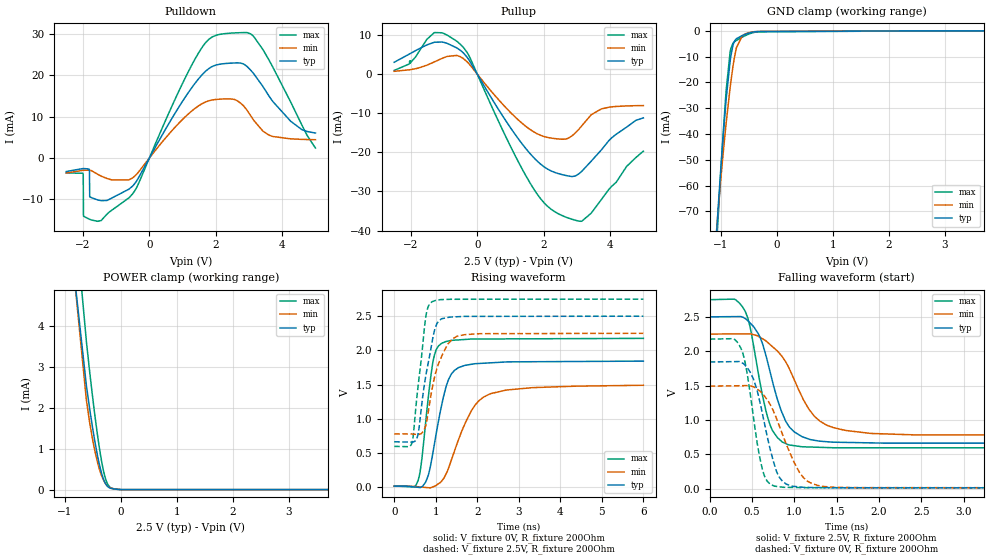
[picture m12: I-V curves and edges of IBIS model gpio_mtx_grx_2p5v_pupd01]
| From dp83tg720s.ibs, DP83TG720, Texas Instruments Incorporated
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[Model]   gpio_mtx_grx_2p5v_pupd01
Model_type   I/O
Polarity   Non-Inverting
Enable   Active-Low
Vinl = 0.75
Vinh = 1.75
Vmeas = 1.25
Vref = 0
Cref = 2pF
Rref = 100000
|   typ   min   max
C_comp   1.19pF   1.18pF   1.2pF
[Voltage Range]   2.5   2.25   2.75
[Temperature Range]   27   150   -40
[Pullup Reference]   2.5   2.25   2.75
[Pulldown Reference]   0   0   0
[Power Clamp Reference]   2.5   2.25   2.75
[GND Clamp Reference]   0   0   0
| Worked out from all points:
|   slope of the pulldown table from 0 to 0.375 V, typ, clamps not added: 69.3 ohm
|   slope of the pullup table from 0 to 0.375 V, typ, clamps not added: 69.5 ohm
|   GND clamp passes 1 mA (typ) near -0.52 V on its own axis
|   POWER clamp passes 1 mA (typ) near -0.44 V on its own axis
|   falling waveform, V_fixture 2.5V, R_fixture 200Ohm: 20-80 % time 264ps typ, 391ps min, 205ps max; typ from 2.5 V to 0.662 V
|   rising waveform, V_fixture 0V, R_fixture 200Ohm: 20-80 % time 357ps typ, 617ps min, 238ps max; typ from 0.013 V to 1.84 V
|   rising waveform, V_fixture 2.5V, R_fixture 200Ohm: 20-80 % time 286ps typ, 362ps min, 225ps max; typ from 0.662 V to 2.5 V
|   falling waveform, V_fixture 0V, R_fixture 200Ohm: 20-80 % time 208ps typ, 303ps min, 161ps max; typ from 1.84 V to 0.013 V
[Pulldown]
|   Voltage   I(typ)   I(min)   I(max)
-2.5V     -3.265mA   -3.621mA   -3.605mA
-2.005V   -2.554mA   -2.975mA   -3.687mA
-1.99V    -2.541mA   -2.964mA   -3.987mA
-1.982V   -2.535mA   -2.958mA   -14.07mA
-1.802V   -2.906mA   -2.952mA   -14.82mA
-1.795V   -9.394mA   -2.961mA   -14.85mA
-1.788V   -9.424mA   -2.97mA    -14.87mA
-617.5mV  -7.551mA   -5.289mA   -9.664mA
1.482V    19.21mA    12.66mA    25.49mA
2.322V    22.93mA    14.34mA    30.18mA
3.147V    20.37mA    9.1mA      29.38mA
5V        6.062mA    4.441mA    2.42mA
[GND Clamp]
|   Voltage   I(typ)   I(min)   I(max)
-2.5V     -617.9mA   -534.4mA   -681.3mA
-1.097V   -85.38mA   -83.09mA   -91.27mA
-1.038V   -65.28mA   -66.86mA   -68.32mA
-962.5mV  -41.99mA   -48.38mA   -41.28mA
-917.5mV  -29.66mA   -38.4mA    -26.83mA
-835mV    -11.96mA   -22.23mA   -8.453mA
-782.5mV  -5.504mA   -13.69mA   -4.805mA
-722.5mV  -3.044mA   -6.63mA    -3.739mA
-617.5mV  -1.829mA   -1.936mA   -2.464mA
-565mV    -1.375mA   -1.221mA   -1.889mA
-302.5mV  -289.6uA   -223.3uA   -396.9uA
5V        0A         0A         0A
[Pullup]
|   Voltage   I(typ)   I(min)   I(max)
-2.5V     3.036mA    720.5uA    942.2uA
-2.042V   5.137mA    1.103mA    2.614mA
-1.3V     8.128mA    3.091mA    10.57mA
-617.5mV  6.711mA    4.78mA     8.425mA
-250mV    3.626mA    2.646mA    4.708mA
852.5mV   -11.84mA   -8.504mA   -15.89mA
1.7V      -21.35mA   -14.76mA   -29.37mA
2.217V    -24.74mA   -16.36mA   -34.52mA
2.848V    -26.19mA   -15.81mA   -37.11mA
3.147V    -24.84mA   -13.2mA    -37.61mA
3.732V    -19.41mA   -8.91mA    -32.11mA
5V        -11.19mA   -8.043mA   -19.7mA
[POWER Clamp]
|   Voltage   I(typ)   I(min)   I(max)
-2.5V     97.53mA    60.54mA    150.4mA
-1.09V    8.453mA    8.804mA    10.81mA
-617.5mV  2.546mA    2.188mA    3.625mA
-565mV    2.037mA    1.696mA    2.964mA
-505mV    1.499mA    1.216mA    2.252mA
-422.5mV  855.7uA    690.1uA    1.37mA
-370mV    524.7uA    436.5uA    888.5uA
-325mV    305.8uA    271.3uA    544.9uA
-280mV    156.5uA    154.6uA    285.8uA
-197.5mV  39.48uA    47.14uA    60.64uA
12.5mV    0A         0A         0A
5V        0A         0A         0A
[Ramp]
R_load = 200
|   typ   min   max
dV/dt_r   1.09795/3.56346e-10   0.886285/6.13825e-10   1.2967/2.36701e-10
dV/dt_f   1.10266/2.61664e-10   0.884047/3.89939e-10   1.29322/2.04854e-10
[Falling Waveform]
V_fixture = 2.5V
V_fixture_min = 2.25V
V_fixture_max = 2.75V
R_fixture = 200Ohm
C_fixture = 0F
|   Time   V(typ)   V(min)   V(max)
0s        2.5V       2.25V      2.75V
289.7ps   2.503V     2.252V     2.758V
411.7ps   2.481V     2.252V     2.599V
476.7ps   2.411V     2.253V     2.355V
581.8ps   2.237V     2.212V     1.629V
702.2ps   1.754V     2.109V     967.7mV
929ps     921mV      1.774V     639.2mV
1.239ns   703.9mV    1.052V     604mV
1.618ns   673mV      845.1mV    595.4mV
6ns       662.2mV    776.4mV    594.6mV
[Rising Waveform]
V_fixture = 0V
V_fixture_min = 0V
V_fixture_max = 0V
R_fixture = 200Ohm
C_fixture = 0F
|   Time   V(typ)   V(min)   V(max)
0s        12.69mV    11.93mV    14.4mV
573ps     -4.336mV   3.092mV    91.58mV
661.7ps   2.918mV    -1.788mV   389.7mV
762.6ps   78.23mV    -7.336mV   976.7mV
926.7ps   482.4mV    840.7uV    1.81V
1.14ns    1.188V     83.97mV    2.102V
1.451ns   1.707V     524.7mV    2.149V
1.894ns   1.8V       1.15V      2.166V
2.291ns   1.817V     1.358V     2.167V
6ns       1.843V     1.489V     2.176V
[Rising Waveform]
V_fixture = 2.5V
V_fixture_min = 2.25V
V_fixture_max = 2.75V
R_fixture = 200Ohm
C_fixture = 0F
|   Time   V(typ)   V(min)   V(max)
0s        662.2mV    776.4mV    594.6mV
431ps     656.4mV    775.3mV    652mV
570.8ps   764.6mV    769.5mV    1.452V
753.3ps   1.599V     885.9mV    2.46V
817.2ps   1.81V      1.086V     2.638V
907.7ps   2.106V     1.421V     2.71V
1.067ns   2.427V     1.805V     2.738V
1.302ns   2.483V     2.098V     2.747V
1.547ns   2.493V     2.213V     2.748V
6ns       2.5V       2.25V      2.75V
[Falling Waveform]
|Gnd
V_fixture = 0V
V_fixture_min = 0V
V_fixture_max = 0V
R_fixture = 200Ohm
C_fixture = 0F
|   Time   V(typ)   V(min)   V(max)
0s        1.843V     1.492V     2.176V
371.5ps   1.841V     1.498V     2.036V
437.7ps   1.766V     1.499V     1.711V
517.3ps   1.595V     1.481V     1.038V
619.5ps   1.112V     1.387V     296mV
761.8ps   359mV      1.104V     37.93mV
861.3ps   105.5mV    786.2mV    21.5mV
1.056ns   26.09mV    245.7mV    16.52mV
1.314ns   15.85mV    37.04mV    14.46mV
6ns       12.69mV    11.93mV    14.4mV
